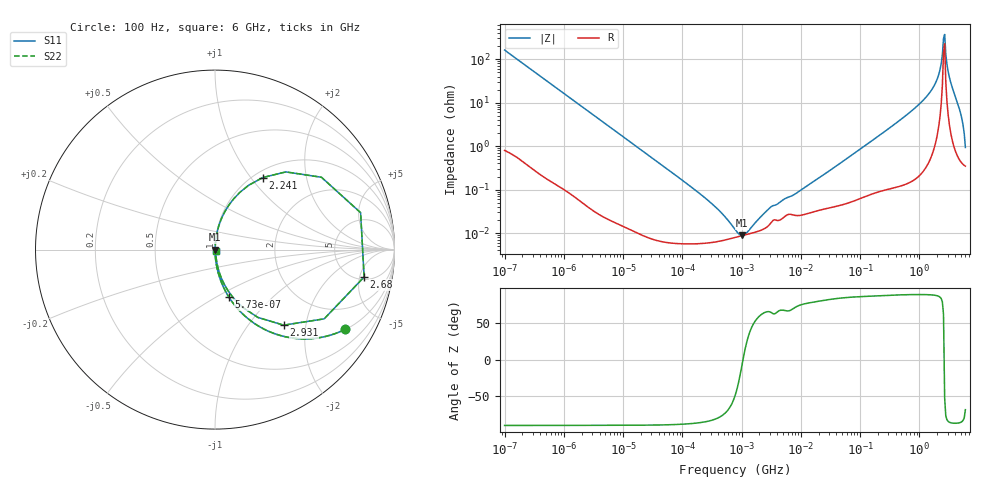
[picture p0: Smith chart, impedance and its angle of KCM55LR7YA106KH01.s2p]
!Murata Part Number: KCM55LR7YA106KH01
!These Parameters are Measured in Series Mode Connection
!Data Generated on Mar 13, 2026
!  o--ll--o
!Port1  Port2
!  o------o
!Operation Temp=25[degC], DC Bias Voltage=0[V]
!Freq. Start=100[Hz] Stop=6[GHz] 401[Steps]
# Hz S RI R 50
!Freq.(Hz) S11(Real) S11(Imag) S21(Real) S21(Imag) S12(Real) S12(Imag) S22(Real) S22(Imag)
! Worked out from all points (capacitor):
!   401 points, 100 Hz to 6 GHz, reference 50 ohm
!   read as one part in series: C = 9.79 uF near 109 Hz
!   lowest |Z| = 8.82 mohm at 1.013 MHz (marker M1)
!   series resonance near 1.058 MHz, so ESL is about 2.3 nH
!   S11 on the Smith chart (normalised r, x): 100 Hz: 1.02, -3.25; 573 Hz: 1.00, -0.57; 2.241 GHz: 1.10, +1.15; 2.68 GHz: 5.52, -5.88; 2.931 GHz: 1.21, -1.51; 6 GHz: 1.01, -0.02
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100  0.724 -0.4446  0.276 0.4446  0.276 0.4446  0.724 -0.4446
205  0.3882 -0.4846  0.6118 0.4846  0.6118 0.4846  0.3882 -0.4846
573  0.0764 -0.2628  0.9236 0.2628  0.9236 0.2628  0.0764 -0.2628
2008  0.00714 -0.0812  0.9929 0.0812  0.9929 0.0812  0.00714 -0.0812
40335  8.25e-05 -0.00411  0.9999 0.00411  0.9999 0.00411  8.25e-05 -0.00411
302498  6.07e-05 -0.000495  0.9999 0.000495  0.9999 0.000495  6.07e-05 -0.000495
774597  7.93e-05 -9.24e-05  0.9999 9.24e-05  0.9999 9.24e-05  7.93e-05 -9.24e-05
1013323  8.73e-05 -1.22e-05  0.9999 1.22e-05  0.9999 1.22e-05  8.73e-05 -1.22e-05
1267578  9.44e-05 5.15e-05  0.9999 -5.15e-05  0.9999 -5.15e-05  9.44e-05 5.15e-05
3103719  0.00017 0.000358  0.9998 -0.000358  0.9998 -0.000358  0.00017 0.000358
1.555665e7  0.000305 0.00143  0.9997 -0.00143  0.9997 -0.00143  0.000305 0.00143
3.124326e8  0.00171 0.0259  0.9983 -0.0259  0.9983 -0.0259  0.00171 0.0259
1.565993e9  0.0379 0.177  0.9621 -0.177  0.9621 -0.177  0.0379 0.177
1.95892e9  0.105 0.2839  0.895 -0.2839  0.895 -0.2839  0.105 0.2839
2.240541e9  0.2667 0.4016  0.7333 -0.4016  0.7333 -0.4016  0.2667 0.4016
2.450438e9  0.5931 0.403  0.4069 -0.403  0.4069 -0.403  0.5931 0.403
2.679998e9  0.8308 -0.1527  0.1692 0.1527  0.1692 0.1527  0.8308 -0.1527
2.931063e9  0.3827 -0.421  0.6173 0.421  0.6173 0.421  0.3827 -0.421
3.205649e9  0.1541 -0.3218  0.8459 0.3218  0.8459 0.3218  0.1541 -0.3218
3.505958e9  0.0721 -0.2285  0.9279 0.2285  0.9279 0.2285  0.0721 -0.2285
4.796499e9  0.00935 -0.0674  0.9906 0.0674  0.9906 0.0674  0.00935 -0.0674
6e9  0.00353 -0.00862  0.9965 0.00862  0.9965 0.00862  0.00353 -0.00862
